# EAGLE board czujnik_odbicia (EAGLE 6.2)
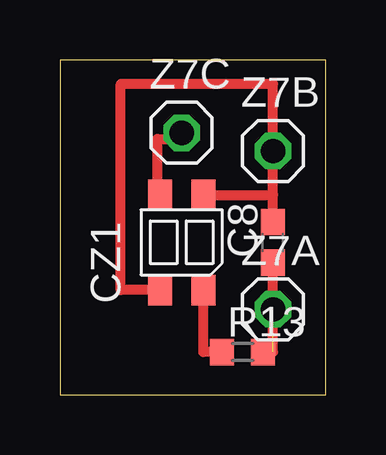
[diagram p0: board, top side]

Size 11.1 x 13.96 mm. Coordinates in mm from the lower left corner, seen from the top.
Outline: 0,0 11.1,0 11.1,13.96 0,13.96 0,0
Copper layers (1*16): Top 0.035mm / dielectric 1.5mm / Bottom 0.035mm
Design rules: minimum track width 10mil, minimum drill 24mil, track to track 8mil, track to pad 8mil, pad to pad 8mil, via to via 8mil, smd to smd 8mil, copper to edge 40mil, drill to drill 8mil, minimum pad ring 10mil, minimum via ring 8mil, stop-mask expansion 4mil, vias tented up to drill 0mil, thermal gap 10mil

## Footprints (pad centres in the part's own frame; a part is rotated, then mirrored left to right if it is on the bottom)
C0603 = smd 1.1 x 1: 1 -0.85,0; 2 0.85,0
TOP = smd 1.27 x 1: ANODA -1.985,-0.9; EMITER -1.985,0.9; KATODA 1.985,-0.9; KOLEKTOR 1.985,0.91
R0603 = smd 1 x 1.1: 1 -0.85,0; 2 0.85,0
1X01 = drill 1.016 octagon: 1 0,0

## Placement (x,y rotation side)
C8  [C0603]  8.89,6.35 90 top
CZ1  KTIR0711S  [TOP]  5.08,6.35 90 top
R13  [R0603]  7.62,1.78 0 top
Z7A  [1X01]  8.89,3.56 0 top
Z7B  [1X01]  8.89,10.16 0 top
Z7C  [1X01]  5.08,10.92 0 top

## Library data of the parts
C8 R13 = rcl
CZ1 = KTIR0711S
Z7A Z7B Z7C = pinhead

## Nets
N$1: CZ1.ANODA R13.1
N$2: C8.2 CZ1.EMITER CZ1.KATODA Z7B.1
N$4: CZ1.KOLEKTOR Z7C.1
N$5: C8.1 R13.2 Z7A.1

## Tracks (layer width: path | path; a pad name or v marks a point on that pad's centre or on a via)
N$1
  Top 0.406: R13.1 5.98,1.78 CZ1.ANODA
N$2
  Top 0.406: C8.2 8.89,8.34 | 8.89,8.34 Z7B.1 8.89,12.95 2.54,12.95 2.54,4.37 CZ1.EMITER | CZ1.KATODA 8.89,8.34
N$4
  Top 0.406: CZ1.KOLEKTOR 4.06,8.34 4.06,10.67 5.08,10.67 Z7C.1
N$5  (1 unrouted)
  Top 0.406: R13.2 8.89,1.78 C8.1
